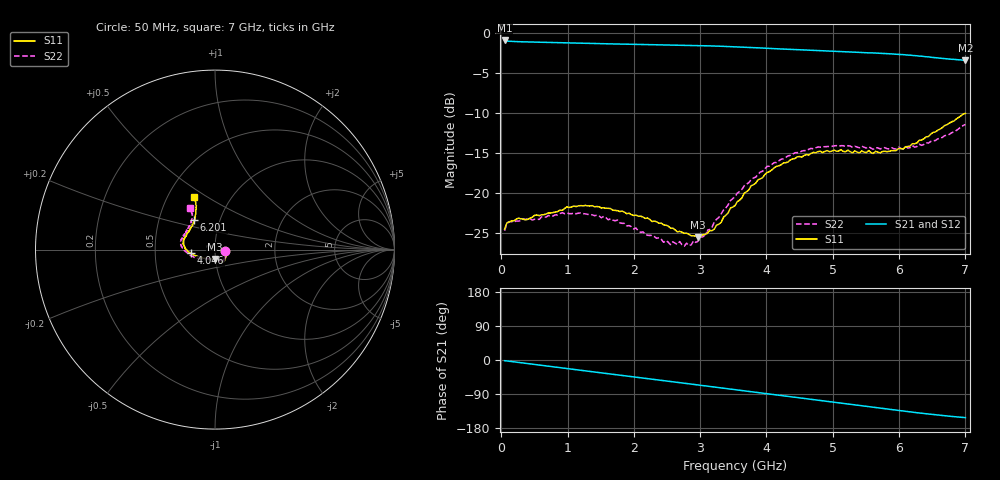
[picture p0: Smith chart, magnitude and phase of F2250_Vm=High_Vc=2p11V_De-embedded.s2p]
! Integrated Device Technology
! Corporate Headquarters
! 6024 Silver Creek Valley Road
! San Jose, CA 95138  USA
! Phone:  1-408-284-8200
! Toll Free:  1-800-223-1366
! Webpage:  http://www.idt.com/
! Timing and RF Division
! 515 Groton Road, Suite 102
! Westford, MA 01886-6024
! Device:  F2250
! Description: Voltage Variable RF Attenuator
! Frequency:  50.0 -  6000.00 MHz
! Package:  3x3 mm Thin QFN Plastic Package: 16 pin
! Ports:  2 RF, 3 DC
!  Pin  1  = GND
!  Pin  2  = NC
!  Pin  3  = RF1  = Port 1
!  Pin  4  = NC
!  Pin  5  = GND
!  Pin  6  = GND
!  Pin  7  = GND
!  Pin  8  = GND
!  Pin  9  = NC
!  Pin 10  = RF2  = Port 2
!  Pin 11  = NC
!  Pin 12  = GND
!  Pin 13  = GND
!  Pin 14  = VCNTRL
!  Pin 15  = VDD
!  Pin 16  = VMODE
! Vcntrl:  2.110 Volts
! Vmode:  +3.300 Volts
! Vdd:  +3.30  Volts
! Current:  1.318 mA
! Data:  The device was measured on a the F2250 evaluation board which has
!  individual transmission lines to the RF pins.  Data was collected
!  using a calibrated network analyzer.  The evaluation board was
!  de-embedded using a TRL calibration technique.
!  The reference plane is the edge of the package pin.
! Misc:  SN 10
!  Action Tracker AT0258
! Date Measured:  2014-11-26
! Date:  2015-10-15  MJV
! Note:
!  Integrated Device Technology supplies this data as a sample of measured
!  data at the package pin for this product.  Your particular data for this
!  product may vary.
!  Data was taken at 25 degrees C.
!  Integrated Device Technology reserves the right to change this data at anytime.
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# GHz S dB R 50
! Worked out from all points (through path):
!   201 points, 50 MHz to 7 GHz, reference 50 ohm
!   highest |S21| = -0.96 dB at 50 MHz (marker M1); lowest = -3.4 dB at 7 GHz (marker M2)
!   group delay of S21, straight-line fit = 61.1 ps
!   lowest |S11| = -25.6 dB at 2.969 GHz (marker M3), VSWR 1.11, Z = 49.6 - j5.24 ohm
!   |S11| at or under -10 dB: start of sweep to end of sweep
!   |S22| runs from -26.7 to -11.5 dB; largest |S21 - S12| = 0.0019
!   S11 on the Smith chart (normalised r, x): 50 MHz: 1.12, -0.02; 4.046 GHz: 0.76, -0.03; 6.201 GHz: 0.75, +0.26; 7 GHz: 0.68, +0.44
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0.05  -24.55 -9.4  -0.96 -1.8  -0.96 -1.8  -24.74 -9.9
0.08475  -23.77 -8.6  -1.03 -2.5  -1.03 -2.5  -23.83 -8.9
0.1195  -23.65 -9.2  -1.06 -3.3  -1.06 -3.2  -23.64 -8.3
0.91875  -22.21 -46.6  -1.25 -21.0  -1.25 -21.1  -22.50 -48.9
1.2315  -21.65 -54.4  -1.32 -27.9  -1.32 -27.9  -22.62 -59.4
1.75275  -22.24 -61.2  -1.41 -39.1  -1.41 -39.1  -23.43 -66.7
2.37825  -23.82 -61.5  -1.50 -52.8  -1.50 -52.8  -25.64 -68.6
2.552  -24.42 -66.0  -1.52 -56.6  -1.52 -56.6  -26.50 -75.1
2.691  -24.84 -73.2  -1.55 -59.7  -1.55 -59.7  -26.11 -82.3
2.7605  -25.08 -75.1  -1.56 -61.3  -1.56 -61.3  -26.69 -86.7
2.969  -25.57 -91.3  -1.60 -65.9  -1.60 -66.0  -26.06 -104.6
3.21225  -24.56 -120.7  -1.66 -71.4  -1.65 -71.5  -23.68 -128.4
3.525  -21.63 -147.5  -1.75 -78.5  -1.75 -78.5  -20.49 -147.1
3.76825  -19.14 -161.0  -1.84 -84.0  -1.84 -84.0  -18.35 -158.3
4.04625  -17.36 -171.0  -1.96 -90.2  -1.96 -90.2  -16.68 -168.9
4.4285  -15.73 178.4  -2.10 -98.6  -2.11 -98.6  -15.00 179.6
4.7065  -14.95 171.2  -2.20 -104.8  -2.20 -104.8  -14.50 173.7
5.054  -14.80 163.0  -2.33 -112.4  -2.33 -112.5  -14.11 166.5
5.85325  -14.83 136.9  -2.63 -129.9  -2.63 -130.1  -14.52 147.6
6.20075  -13.87 125.0  -2.84 -137.7  -2.84 -137.8  -14.12 138.5
6.54825  -12.40 116.7  -3.11 -144.7  -3.11 -144.8  -13.47 127.1
7  -10.08 111.7  -3.44 -152.0  -3.44 -152.1  -11.47 120.9
